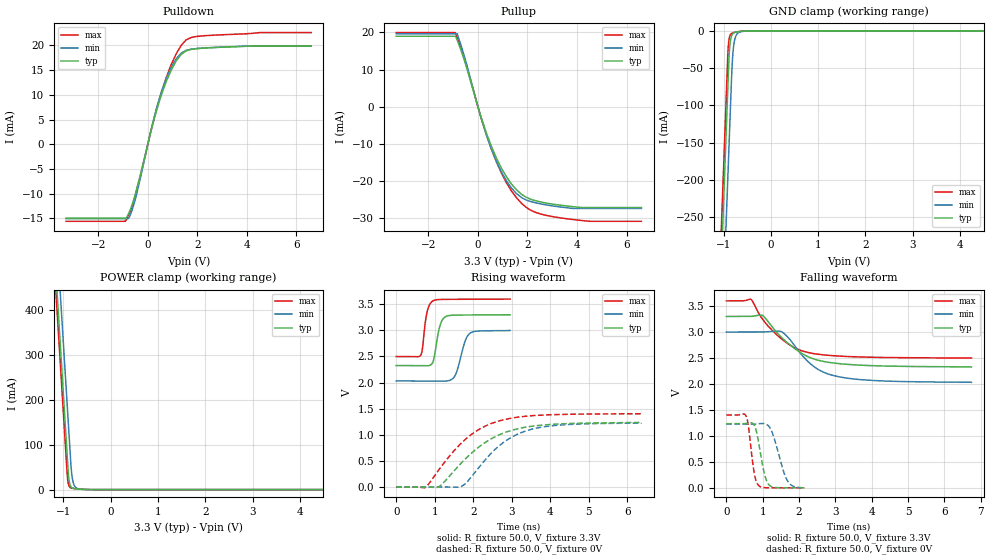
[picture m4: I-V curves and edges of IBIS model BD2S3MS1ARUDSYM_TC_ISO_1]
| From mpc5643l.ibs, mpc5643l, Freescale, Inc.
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| *** New cell (Generated with 5.14beta1 (Sep 20 2010 13:23:23))
[Model]   BD2S3MS1ARUDSYM_TC_ISO_1
Model_type I/O
Polarity   Non-Inverting
Enable   Active-Low
| CAP_THRESHOLD on pad pad is "CMOS" :
| Rising=10.0% of VDDE1   Falling=90.0% of VDDE1
| C_comp min and max val. don't necessarily correlate with the min and max pvt
| but are the smallest and greatest pad capacitance found.
| var   typ   min   max
C_comp   1.90207pF  1.77304pF  2.06246pF
Vinl = 1.05V | Dummy value overriden by next lines
Vinh = 2.34V | Dummy value overriden by next lines
Vmeas = 1.65V   | Reference voltage for timing measurements
Cref  = 25.0pF   | Timing specification test load capacitance value
Rref  = 1.0MOhm   | Timing specification test load resistance value
Vref  = 1.65V   | Timing specification test load voltage
[Model Spec]
| TIME_THRESHOLD on pin ipp_ind is "CORE" :
| Rising=40.0% of VDD   Falling=60.0% of VDD
Vinl 1.30950V 1.19650V 1.40650V
Vinh 1.89650V 1.72150V 2.04550V
| variable   typ   min   max
[Temperature Range] 25.0 150.0 -40.0
| variable   typ   min   max
[Voltage Range] 3.3V 3.0V 3.6V
| variable   typ   min   max
[POWER Clamp Reference] 3.3V 3.0V 3.6V
| variable   typ   min   max
[GND Clamp Reference] 0V 0V 0V
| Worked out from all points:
|   slope of the pulldown table from 0 to 0.495 V, typ, clamps not added: 54.3 ohm
|   slope of the pullup table from 0 to 0.495 V, typ, clamps not added: 50.6 ohm
|   GND clamp passes 1 mA (typ) near -0.67 V on its own axis
|   POWER clamp passes 1 mA (typ) near -0.66 V on its own axis
|   rising waveform, R_fixture 50.0, V_fixture 3.3V: 20-80 % time 145ps typ, 216ps min, 118ps max; typ from 2.33 V to 3.3 V
|   falling waveform, R_fixture 50.0, V_fixture 3.3V: 20-80 % time 1.01ns typ, 877ps min, 944ps max; typ from 3.3 V to 2.33 V
|   rising waveform, R_fixture 50.0, V_fixture 0V: 20-80 % time 1.21ns typ, 1.06ns min, 1.14ns max; typ from 0 V to 1.24 V
|   falling waveform, R_fixture 50.0, V_fixture 0V: 20-80 % time 198ps typ, 305ps min, 147ps max; typ from 1.24 V to 0 V
[POWER Clamp]
-3.3V     4.125A     4.239A     4.084A
-1.21V    572.2mA    686.2mA    530.8mA
-1.14V    453.2mA    567.2mA    411.8mA
-1.07V    334.2mA    448.2mA    292.8mA
-1V       215.2mA    329.2mA    173.8mA
-910mV    62.21mA    176.2mA    24.61mA
-880mV    22.38mA    125.2mA    8.495mA
-840mV    6.765mA    57.19mA    3.971mA
-810mV    3.645mA    26.2mA     3.059mA
-770mV    2.237mA    9.849mA    2.403mA
-610mV    694.5uA    892.2uA    750.7uA
6.6V      0A         0A         0A
[GND Clamp]
-3.3V     -4.141A    -4.261A    -4.096A
-1.08V    -366.9mA   -487.3mA   -321.6mA
-910mV    -77.88mA   -198.3mA   -32.59mA
-890mV    -43.88mA   -164.3mA   -14.43mA
-870mV    -21.84mA   -130.3mA   -7.503mA
-850mV    -11.54mA   -96.29mA   -4.735mA
-830mV    -6.662mA   -62.29mA   -3.515mA
-810mV    -4.283mA   -37.08mA   -2.874mA
-780mV    -2.674mA   -17.5mA    -2.282mA
-740mV    -1.782mA   -6.992mA   -1.702mA
-540mV    -228.3uA   -504.1uA   -137.1uA
6.6V      5.454nA    1.731uA    35.72pA
| variable   typ   min   max
[Pullup Reference] 3.3V 3.0V 3.6V
| variable   typ   min   max
[Pulldown Reference] 0V 0V 0V
[Pullup]
-3.3V     18.95mA    19.62mA    19.93mA
-920mV    18.95mA    19.62mA    19.93mA
-840mV    17.95mA    19.62mA    18.61mA
-710mV    15.65mA    17.05mA    16.29mA
-470mV    10.79mA    11.73mA    11.3mA
140mV     -3.061mA   -3.283mA   -3.266mA
740mV     -13.7mA    -14.6mA    -14.74mA
1.35V     -20.74mA   -21.83mA   -22.6mA
1.96V     -24.37mA   -25.1mA    -27.1mA
2.57V     -25.66mA   -26.17mA   -28.91mA
3.78V     -26.83mA   -27.31mA   -30.28mA
6.6V      -27.1mA    -27.34mA   -30.8mA
[Pulldown]
-3.3V     -14.94mA   -15.06mA   -15.58mA
-890mV    -14.94mA   -15.06mA   -15.46mA
-740mV    -13.62mA   -14.67mA   -13.92mA
-550mV    -10.92mA   -11.95mA   -11.15mA
-270mV    -5.613mA   -6.208mA   -5.736mA
140mV     2.888mA    3.121mA    2.995mA
340mV     6.607mA    7.074mA    6.906mA
740mV     12.63mA    13.26mA    13.43mA
1.15V     16.87mA    17.3mA     18.32mA
1.55V     18.91mA    19mA       21.12mA
2.5V      19.51mA    19.53mA    22.02mA
6.6V      19.9mA     19.82mA    22.59mA
[Ramp]
dV/dt_r 740.93046mV/1.21456ns 735.03082mV/1.05704ns 841.42446mV/1.13895ns
dV/dt_f 584.0842mV/1.00946ns 581.49511mV/876.52826ps 660.6039mV/943.97177ps
R_load = 50.0
| Removed startup time: 0s 0s 0s  .
| Removed end time: 2.955ns.
[Rising Waveform]
R_fixture   = 50.0
V_fixture   = 3.3V
V_fixture_min = 3.0V
V_fixture_max = 3.6V
0s        2.327V     2.031V     2.499V
637ps     2.327V     2.031V     2.524V
800ps     2.322V     2.031V     3.349V
966ps     2.42V      2.031V     3.571V
1.125ns   3.06V      2.03V      3.593V
1.263ns   3.255V     2.027V     3.595V
1.531ns   3.293V     2.137V     3.597V
1.779ns   3.296V     2.775V     3.597V
1.908ns   3.296V     2.942V     3.598V
2.957ns   3.3V       3V         3.6V
| Removed startup time: 0s 0s 0s  .
| Removed end time: 6.741ns.
[Falling Waveform]
R_fixture   = 50.0
V_fixture   = 3.3V
V_fixture_min = 3.0V
V_fixture_max = 3.6V
0s        3.3V       3V         3.6V
681ps     3.301V     3V         3.631V
999ps     3.319V     3.001V     3.245V
1.497ns   2.913V     3.013V     2.88V
1.71ns    2.776V     2.889V     2.768V
2.22ns    2.534V     2.451V     2.61V
2.457ns   2.471V     2.311V     2.579V
2.718ns   2.428V     2.214V     2.557V
3.414ns   2.373V     2.104V     2.526V
6.747ns   2.327V     2.031V     2.499V
| Removed startup time: 0s 0s 0s  .
| Removed end time: 6.36ns.
[Rising Waveform]
R_fixture   = 50.0
V_fixture   = 0V
V_fixture_min = 0V
V_fixture_max = 0V
0s        11.74nV    645.5nV    11.16nV
759ps     227.3uV    -1.454uV   -8.088mV
1.119ns   8.223mV    413.9uV    341.8mV
1.683ns   452.6mV    7.286mV    833.2mV
1.833ns   563.6mV    87.83mV    935.1mV
2.127ns   753.5mV    354.1mV    1.092V
2.604ns   974.4mV    744.5mV    1.249V
3.141ns   1.112V     1.007V     1.335V
3.81ns    1.185V     1.15V      1.378V
6.366ns   1.235V     1.225V     1.402V
| Removed startup time: 0s 0s 0s  .
| Removed end time: 2.144ns.
[Falling Waveform]
R_fixture   = 50.0
V_fixture   = 0V
V_fixture_min = 0V
V_fixture_max = 0V
0s        1.235V     1.225V     1.402V
548ps     1.241V     1.225V     1.376V
612ps     1.251V     1.225V     1.169V
770ps     1.205V     1.227V     273.6mV
889ps     873.2mV    1.234V     43.92mV
1.054ns   255.8mV    1.235V     4.455mV
1.186ns   49.96mV    1.171V     1.449mV
1.668ns   1.014mV    153.8mV    564.1uV
1.82ns    783.9uV    37.44mV    502.2uV
2.146ns   62.25uV    95.45uV    37.81uV
